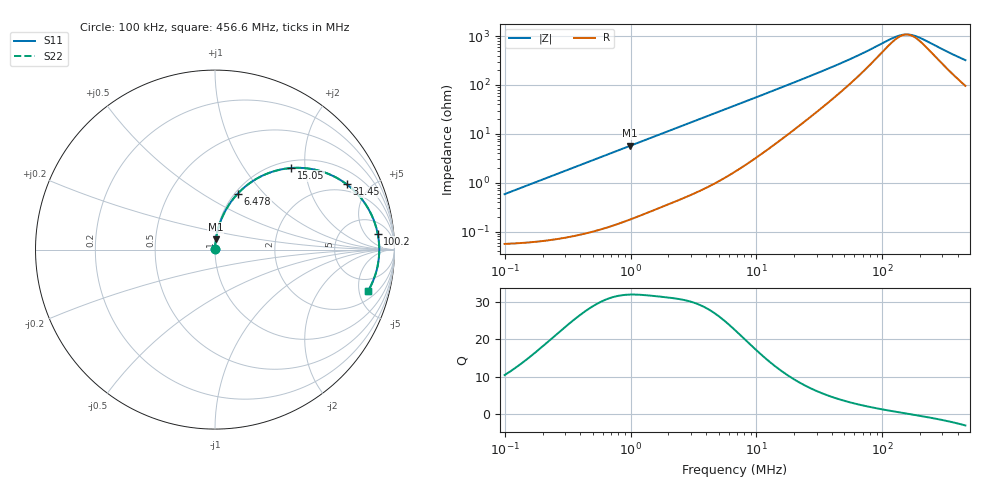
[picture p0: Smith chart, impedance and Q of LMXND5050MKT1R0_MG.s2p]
! LMXND5050MKT1R0_MG  S-PARAMETER MODEL  ( General Type )
! Model Generated by TAIYO YUDEN Corporation (https://www.yuden.co.jp/en/)
! Version 1.0
! TAIYO YUDEN Control No. 191023NI43SB-FBB
! Copyright(c) 2019 TAIYO YUDEN CO.,LTD. All Rights Reserved.
! Product Description (link to TY-COMPAS)
! https://ds.yuden.co.jp/TYCOMPAS/or/detail?pn=LMXND5050MKT1R0NMG&u=M
! Products Name : Inductors
! Characteristics :
!  Inductance : 1.0 uH , SRF(min) : 100 MHz , DC Resistance(max) : 0.0636 Ohm
!  Rated Current : Saturation :4500 mA , Temp Rise : 2300 mA (40 degC)
!  Case Size : 4.9 x 4.9 / 0.193 x 0.193 [mm/inch] , Thickness : 1.2 / 0.047 [mm/inch]
!  (Conditions: Temperature = 25 degC , DC Bias Current/Voltage = 0A / 0V)
! External Node Assignments :
!  1  o---GGG---o  2
! GND o---------o GND
! Frequency Range : 0.1MHz  -  456.598367MHz  [ 402 STEP ]
# MHz S RI R 50
! Freq[MHz].  S11 Real  S11 Imag  S21 Real  S21 Imag  S12 Real  S12 Imag  S22 Real  S22 Imag
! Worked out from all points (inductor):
!   401 points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, 100 kHz to 456.6 MHz, reference 50 ohm
!   read as one part in series: L = 928 nH near 104.3 kHz
!   highest Q = 32.1 at 993.6 kHz (marker M1), where L = 913 nH
!   self-resonance near 155.8 MHz
!   S11 on the Smith chart (normalised r, x): 100 kHz: 1.00, +0.01; 6.478 MHz: 1.03, +0.73; 15.05 MHz: 1.14, +1.69; 31.45 MHz: 1.61, +3.57; 100.2 MHz: 11, +11; 456.6 MHz: 2.92, -6.14
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0.1  0.000596 0.00583  0.9994 -0.00583  0.9994 -0.00583  0.000596 0.00583
0.410178  0.00144 0.0237  0.9986 -0.0237  0.9986 -0.0237  0.00144 0.0237
0.993626  0.00499 0.0566  0.995 -0.0566  0.995 -0.0566  0.00499 0.0566
1.682457  0.012 0.0943  0.988 -0.0943  0.988 -0.0943  0.012 0.0943
3.746276  0.049 0.1992  0.951 -0.1992  0.951 -0.1992  0.049 0.1992
6.478426  0.1274 0.3125  0.8726 -0.3125  0.8726 -0.3125  0.1274 0.3125
6.901063  0.1416 0.3269  0.8584 -0.3269  0.8584 -0.3269  0.1416 0.3269
9.872934  0.248 0.4038  0.752 -0.4038  0.752 -0.4038  0.248 0.4038
15.04607  0.4248 0.4545  0.5752 -0.4545  0.5752 -0.4545  0.4248 0.4545
20.20722  0.5608 0.4444  0.4392 -0.4444  0.4392 -0.4444  0.5608 0.4444
27.71655  0.69 0.3931  0.31 -0.3931  0.31 -0.3931  0.69 0.3931
31.45084  0.7329 0.3646  0.2671 -0.3646  0.2671 -0.3646  0.7329 0.3646
40.49657  0.8015 0.3012  0.1985 -0.3012  0.1985 -0.3012  0.8015 0.3012
53.25411  0.8524 0.2308  0.1476 -0.2308  0.1476 -0.2308  0.8524 0.2308
100.1886  0.9069 0.0867  0.0931 -0.0867  0.0931 -0.0867  0.9069 0.0867
113.6871  0.9111 0.0612  0.0889 -0.0612  0.0889 -0.0612  0.9111 0.0612
143.3337  0.9149 0.016  0.0851 -0.016  0.0851 -0.016  0.9149 0.016
159.2548  0.9152 -0.0042  0.0848 0.0042  0.0848 0.0042  0.9152 -0.0042
176.9444  0.9146 -0.0245  0.0854 0.0245  0.0854 0.0245  0.9146 -0.0245
209.4245  0.9116 -0.0574  0.0884 0.0574  0.0884 0.0574  0.9116 -0.0574
293.3653  0.8972 -0.1271  0.1028 0.1271  0.1028 0.1271  0.8972 -0.1271
456.5984  0.8524 -0.2314  0.1476 0.2314  0.1476 0.2314  0.8524 -0.2314
